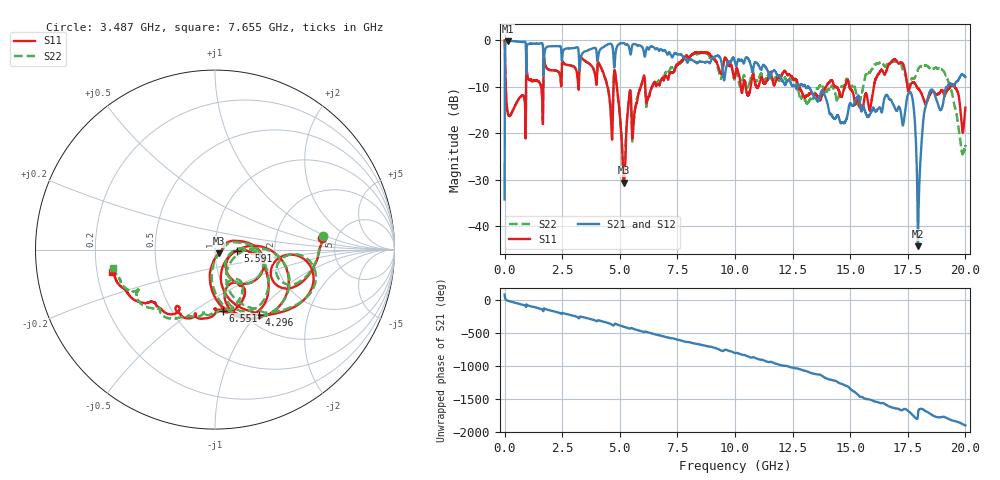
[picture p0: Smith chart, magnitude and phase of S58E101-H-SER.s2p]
!{S58E101}
!Johanson Technology Inc.
!www.johansontechnology.com
!Test Board Conditions:
!Substrate Type  RO4350B
!Substrate Thickness  60 mil
!Substrate Dk  3.66
!TL Type: GCPW
!TL Trace Width  115 mil
!TL Gap  52 mil
!Electrode orientation  Horizontal
!DUT TOPOLOGY	SERIES
!Mounting Pad LxW  55x428 mil
! Created Tue Apr 13 22:45:40 2021
# mhz S ma R 50
! 2 Port Network Data from SP1.SP block
! freq  magS11  angS11  magS21  angS21  magS12  angS12  magS22  angS22
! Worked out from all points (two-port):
!   20001 points, 300 kHz to 20 GHz, reference 50 ohm
!   highest |S21| = -0.11 dB at 160.3 MHz (marker M1); lowest = -44.4 dB at 17.94 GHz (marker M2)
!   |S21| within 3 dB of the highest: 4.807 GHz to 6.063 GHz (1.255 GHz wide, 23.1 % of centre); 6.107 GHz to 7.209 GHz (1.102 GHz wide, 16.6 % of centre)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
!   lowest |S11| = -30.7 dB at 5.175 GHz (marker M3), VSWR 1.06, Z = 52 - j2.19 ohm
!   |S11| at or under -10 dB: 12.76 GHz to 13.95 GHz (1.188 GHz wide, 8.89 % of centre); 14.97 GHz to 16.03 GHz (1.059 GHz wide, 6.83 % of centre); 17.89 GHz to 19.34 GHz (1.453 GHz wide, 7.8 % of centre)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
!   |S22| runs from -30.2 to 0.0 dB; largest |S21 - S12| = 0.0086
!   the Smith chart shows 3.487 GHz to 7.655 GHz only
!   S11 on the Smith chart (normalised r, x): 3.487 GHz: 3.85, +0.77; 4.296 GHz: 1.15, -1.03; 5.591 GHz: 1.28, -0.02; 6.551 GHz: 0.86, -0.66; 7.655 GHz: 0.26, -0.10
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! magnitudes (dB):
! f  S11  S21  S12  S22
! 300 kHz  0.0  -34.3  -34.3  0.0
! 160.3 MHz  -16.1  -0.1  -0.1  -16.0
! 3.334 GHz  -3.7  -3.3  -3.3  -3.7
! 3.487 GHz  -4.4  -2.4  -2.4  -4.4
! 4.296 GHz  -7.2  -1.5  -1.5  -7.2
! 4.616 GHz  -16.4  -0.8  -0.8  -15.8
! 4.837 GHz  -8.5  -2.0  -2.0  -8.4
! 5.175 GHz  -30.7  -0.6  -0.6  -29.9
! 5.396 GHz  -12.7  -1.4  -1.4  -12.6
! 5.591 GHz  -18.1  -0.8  -0.8  -18.2
! 6.551 GHz  -9.3  -1.9  -1.9  -9.3
! 6.667 GHz  -9.5  -2.0  -2.0  -8.8
! 7.655 GHz  -4.6  -3.0  -3.0  -4.8
! 10 GHz  -7.8  -4.7  -4.7  -8.0
! 13.33 GHz  -11.5  -11.1  -11.1  -12.7
! 15.85 GHz  -15.0  -16.0  -15.9  -6.9
! 16.67 GHz  -5.2  -12.4  -12.4  -4.8
! 17.65 GHz  -9.3  -11.5  -11.5  -8.4
! 17.94 GHz  -10.3  -44.4  -44.5  -6.4
! 18.44 GHz  -11.8  -11.3  -11.2  -6.0
! 19.17 GHz  -11.1  -10.2  -10.2  -7.8
! 20 GHz  -14.5  -7.9  -7.8  -22.6
